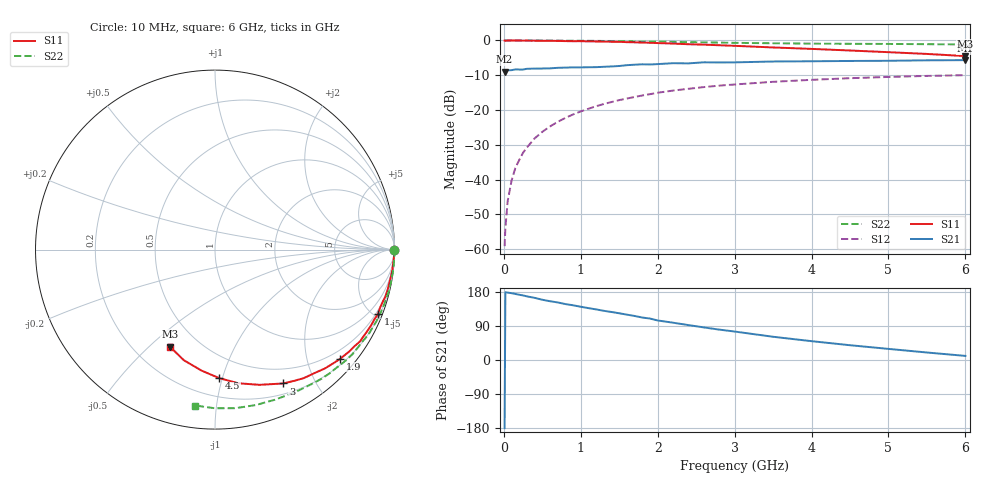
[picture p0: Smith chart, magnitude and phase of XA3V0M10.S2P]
! SIEMENS Discrete & RF Semiconductors
! BFY180
! Si NPN RF Bipolar Junction Transistor in MICRO-X
! VCE = 3 V  IC = 0.1 mA
! Common Emitter S-Parameters:  May  1997
# GHz  S  MA  R  50
!  f  S11  S21  S12  S22
! GHz  MAG  ANG  MAG  ANG  MAG  ANG  MAG  ANG
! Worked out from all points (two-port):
!   36 points, 10 MHz to 6 GHz, reference 50 ohm
!   highest |S21| = -5.66 dB at 6 GHz (marker M1); lowest = -9.0 dB at 10 MHz (marker M2)
!   |S21| within 3 dB of the highest: 19.19 MHz to end of sweep
!   lowest |S11| = -4.5 dB at 6 GHz (marker M3), VSWR 3.95, Z = 17.4 - j29.1 ohm
!   |S11| at or under -10 dB: nowhere
!   |S22| runs from -1.2 to 0.0 dB; largest |S21 - S12| = 0.39
!   S11 on the Smith chart (normalised r, x): 10 MHz: open; 1 GHz: 0.35, -5.25; 1.9 GHz: 0.31, -2.64; 3 GHz: 0.32, -1.59; 4.5 GHz: 0.33, -0.98; 6 GHz: 0.35, -0.58
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0.01  0.996 -0.2  0.356 -179.8  0.0011 83.5  0.9999 0.0
0.02  0.9914 -0.4  0.37 178.9  0.002 87.8  0.9999 -0.4
0.05  0.9954 -0.8  0.372 177.9  0.0049 88.8  0.9999 -0.9
0.1  0.9981 -2.0  0.374 176.3  0.0096 88.3  0.9999 -1.9
0.15  0.9971 -3.2  0.383 174.3  0.0147 88.1  0.9999 -2.9
0.25  0.9943 -5.6  0.382 170.4  0.0243 85.4  0.9999 -4.8
0.4  0.9914 -8.7  0.394 164.0  0.039 82.1  0.9982 -7.5
0.5  0.9887 -10.7  0.395 159.0  0.0485 80.4  0.9976 -9.4
0.7  0.9848 -15.4  0.404 151.9  0.0675 76.0  0.9955 -13.3
1  0.9761 -21.5  0.41 140.5  0.0953 69.9  0.9899 -19.0
1.1  0.9694 -23.6  0.412 136.9  0.1041 68.0  0.9876 -20.8
1.5  0.9564 -32.3  0.429 123.3  0.1387 59.8  0.9777 -28.3
1.8  0.9314 -39.2  0.454 112.1  0.1617 54.4  0.966 -33.7
1.9  0.9261 -41.0  0.451 109.4  0.1688 52.3  0.9639 -35.5
2  0.9168 -43.2  0.457 104.3  0.177 50.5  0.9624 -37.2
2.2  0.9022 -47.2  0.471 98.4  0.1903 46.6  0.9544 -40.8
2.6  0.8703 -55.4  0.485 86.0  0.2134 39.5  0.9394 -47.4
3  0.837 -63.0  0.484 75.1  0.2327 32.7  0.9238 -53.8
3.5  0.7931 -71.8  0.498 61.3  0.2542 25.5  0.911 -61.0
4.5  0.7169 -88.0  0.507 39.0  0.2865 11.7  0.8953 -75.4
5.5  0.64 -105.8  0.518 19.8  0.309 -1.3  0.8839 -90.1
6  0.5958 -115.0  0.521 10.8  0.3167 -8.0  0.8757 -97.3
